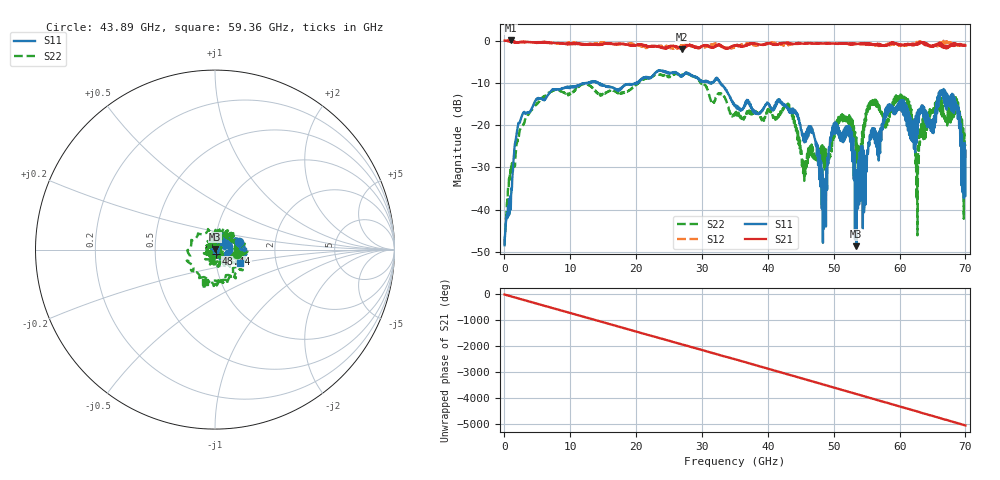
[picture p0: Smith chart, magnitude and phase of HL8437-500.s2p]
! 7/8/2021 2:59:28 PM
! H:\PROTOTYPE_DATA\DCBS_7-8-21\500NF_50V_CERAMIC_1.S2P
! CHANNEL.1
! TR.MEASUREMENT
! CORRECTED.DATA
# GHZ S RI R 50.0
! FREQ.GHZ  S11RE  S11IM  S21RE  S21IM  S12RE  S12IM  S22RE  S22IM
!; PortSelection: Port_12
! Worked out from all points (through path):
!   2000 points, 35 MHz to 70 GHz, reference 50 ohm
!   highest |S21| = 0.03 dB at 1.015 GHz (marker M1); lowest = -2.0 dB at 26.95 GHz (marker M2)
!   group delay of S21, straight-line fit = 200 ps
!   lowest |S11| = -48.7 dB at 53.45 GHz (marker M3), VSWR 1.01, Z = 49.8 + j0.292 ohm
!   |S11| at or under -10 dB: start of sweep to 12.65 GHz; 14.2 GHz to 20.04 GHz (5.841 GHz wide, 34.1 % of centre); 32.8 GHz to end of sweep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
!   |S22| runs from -48.3 to -7.6 dB; largest |S21 - S12| = 0.19
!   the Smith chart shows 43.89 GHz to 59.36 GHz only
!   S11 on the Smith chart (normalised r, x): 43.89 GHz: 1.31, +0.11; 48.44 GHz: 1.01, -0.05; 59.36 GHz: 1.30, -0.20
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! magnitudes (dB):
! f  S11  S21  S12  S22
! 35 MHz  -48.4  0.0  0.0  -48.3
! 1.015 GHz  -36.5  0.0  -0.1  -29.5
! 2.765 GHz  -17.5  -0.4  -0.3  -20.1
! 11.72 GHz  -10.2  -0.9  -0.9  -10.4
! 23.38 GHz  -7.1  -1.4  -1.2  -8.0
! 26.95 GHz  -8.4  -2.0  -1.2  -8.3
! 35.03 GHz  -15.2  -1.1  -1.6  -17.1
! 43.89 GHz  -17.0  -0.8  -0.8  -17.9
! 45.5 GHz  -22.2  -0.7  -0.6  -31.2
! 46.69 GHz  -21.8  -0.7  -0.6  -25.7
! 48.44 GHz  -32.6  -0.7  -0.7  -25.1
! 50.23 GHz  -19.5  -0.7  -0.8  -21.1
! 52.43 GHz  -20.4  -0.7  -0.8  -20.3
! 53.45 GHz  -48.7  -0.8  -0.8  -23.0
! 55.72 GHz  -22.0  -0.7  -1.1  -14.4
! 58.34 GHz  -16.9  -0.8  -1.1  -18.7
! 59.36 GHz  -16.1  -0.8  -0.9  -14.3
! 61.46 GHz  -22.4  -0.9  -0.9  -14.4
! 62.58 GHz  -24.0  -0.9  -0.8  -37.6
! 65.91 GHz  -14.6  -0.8  -1.3  -13.1
! 68.46 GHz  -16.3  -1.1  -1.1  -16.3
! 70 GHz  -26.1  -1.2  -1.1  -24.6
